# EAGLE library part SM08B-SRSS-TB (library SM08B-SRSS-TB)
Connector Header Surface Mount, Right Angle 8 position 0.039" (1.00mm) Source: Datasheet
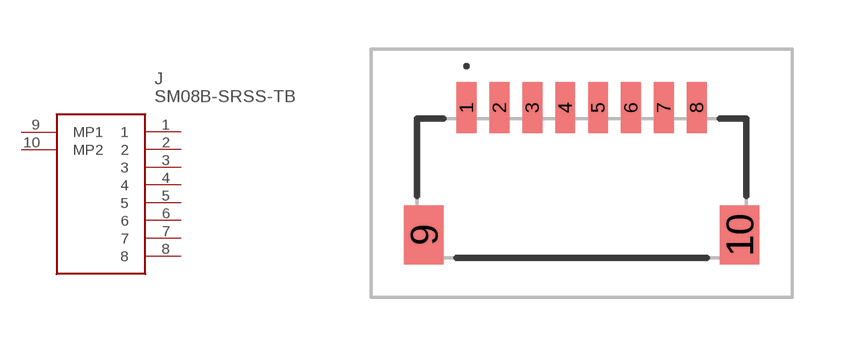
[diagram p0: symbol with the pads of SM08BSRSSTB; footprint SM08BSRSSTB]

Designator prefix J

## SM08B-SRSS-TB (Description: Connector Header Surface Mount, Right Angle 8 position 0.039" (1.00mm); Height: 2.95mm; Manufacturer_Name: JST (JAPAN SOLDERLESS TERMINALS); Manufacturer_Part_Number: SM08B-SRSS-TB; Mouser_Part_Number: N/A; Mouser_Price-Stock: https://www.mouser.co.uk/ProductDetail/JST-Commercial/SM08B-SRSS-TB?qs=IKkN%2F947nfBrj0Hsszhebg%3D%3D)  [SM08BSRSSTB]
1  1
2  2
3  3
4  4
5  5
6  6
7  7
8  8
9  MP1
10  MP2

## Footprint SM08BSRSSTB (pad centres in mm)
SM08B-SRSS-TB-1
smd 0.6 x 1.55: 1 -3.5,2.288; 2 -2.5,2.288; 3 -1.5,2.288; 4 -0.5,2.288; 5 0.5,2.288; 6 1.5,2.288; 7 2.5,2.288; 8 3.5,2.288
smd 1.2 x 1.8: 9 -4.8,-1.588; 10 4.8,-1.588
